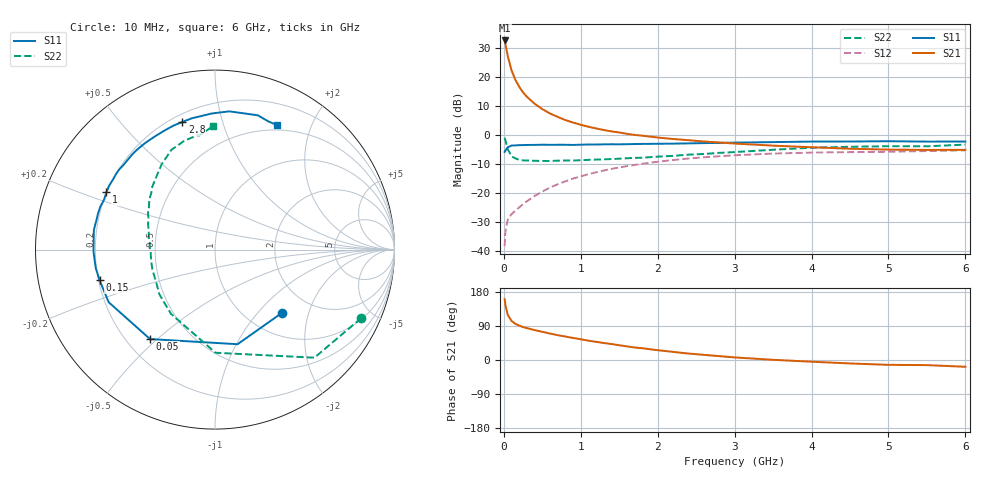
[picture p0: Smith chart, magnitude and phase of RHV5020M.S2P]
! SIEMENS Small Signal Semiconductors
! BFR106
! Si NPN RF Bipolar Junction Transistor in SOT23
! VCE = 0.5 V  IC = 20 mA
! Common Emitter S-Parameters:  August  1996
# GHz  S  MA  R  50
!  f  S11  S21  S12  S22
! GHz  MAG  ANG  MAG  ANG  MAG  ANG  MAG  ANG
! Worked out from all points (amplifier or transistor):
!   36 points, 10 MHz to 6 GHz, reference 50 ohm
!   highest |S21| = 32.6 dB at 10 MHz (marker M1)
!   |S21| within 3 dB of that: start of sweep to 33.21 MHz
!   unconditionally stable (mu >= 1): 302.1 MHz to end of sweep
!   at 250 MHz: K = 0.94, MSG = 19.2 dB, |S12| = -23.8 dB
!   at 1.4 GHz: K = 1.11, MAG = 4.5 dB, |S12| = -11.6 dB
!   at 6 GHz: K = 1.03, MAG = -1.0 dB, |S12| = -5.2 dB
!   S11 on the Smith chart (normalised r, x): 10 MHz: 1.43, -1.37; 50 MHz: 0.29, -0.47; 150 MHz: 0.20, -0.13; 1 GHz: 0.20, +0.24; 2.8 GHz: 0.24, +0.75; 6 GHz: 0.44, +1.52
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0.01  0.5136 -43.2  42.81 160.6  0.0122 75.5  0.8999 -25.1
0.02  0.542 -76.6  37.43 145.5  0.0217 62.2  0.8183 -47.4
0.05  0.616 -126.0  23.18 119.4  0.0349 45.0  0.5748 -89.7
0.1  0.661 -153.7  13.1 103.1  0.0435 42.2  0.4339 -124.4
0.15  0.6652 -165.1  8.957 95.4  0.0497 45.0  0.3974 -141.4
0.2  0.6723 -171.2  6.815 90.7  0.0569 48.8  0.3742 -151.1
0.25  0.6738 -176.1  5.448 86.9  0.0648 51.9  0.3674 -158.5
0.3  0.6772 -179.1  4.578 84.1  0.0726 54.6  0.3654 -162.9
0.4  0.6786 174.7  3.477 78.9  0.0894 57.7  0.3611 -169.9
0.5  0.6837 170.7  2.808 74.4  0.1066 59.3  0.3591 -174.7
0.6  0.6805 166.3  2.362 69.8  0.1246 59.7  0.3584 -178.0
0.8  0.682 159.3  1.819 61.9  0.1601 59.0  0.3652 176.1
1  0.6842 152.1  1.508 54.7  0.1951 57.0  0.3691 171.5
1.1  0.6891 148.9  1.395 51.0  0.2121 55.7  0.375 169.4
1.3  0.6937 142.6  1.223 44.8  0.2456 52.7  0.382 164.8
1.6  0.6978 134.1  1.053 36.0  0.2921 47.9  0.3996 159.0
2.2  0.7135 118.5  0.858 21.4  0.3728 37.4  0.4392 146.8
2.8  0.7341 104.4  0.748 10.2  0.4326 27.2  0.4949 134.9
3.5  0.7584 91.4  0.659 0.5  0.481 16.2  0.5596 122.2
4.5  0.7762 77.8  0.583 -9.1  0.509 2.7  0.6299 105.7
5.5  0.7735 67.4  0.556 -13.5  0.5319 -5.3  0.642 97.9
6  0.7751 63.6  0.558 -17.9  0.5466 -11.4  0.6861 91.1
